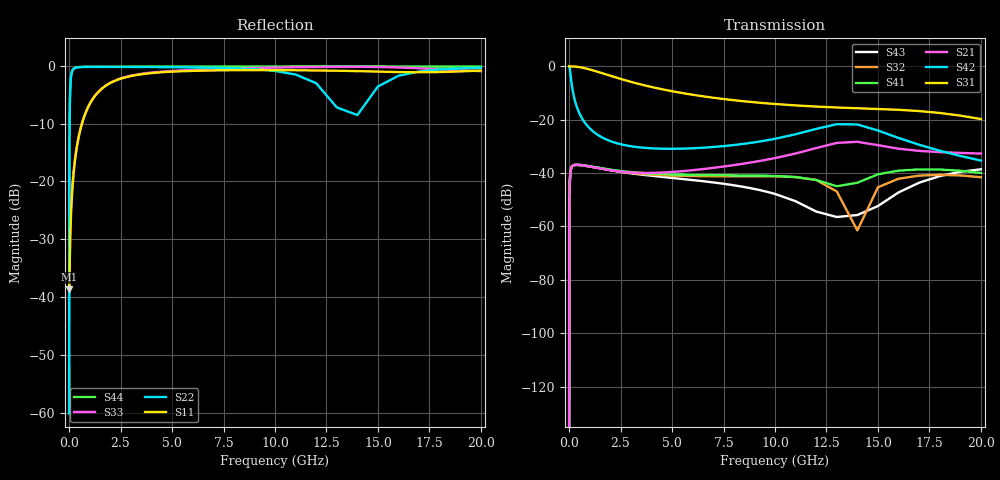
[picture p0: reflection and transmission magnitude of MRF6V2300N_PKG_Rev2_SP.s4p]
! Created Fri Apr 13 13:24:45 2007
# mhz S ma R 50
! 4 Port Network Data from SP1.SP block
! freq  magS11  angS11  magS12  angS12  magS13  angS13  magS14  angS14
!  magS21  angS21  magS22  angS22  magS23  angS23  magS24  angS24
!  magS31  angS31  magS32  angS32  magS33  angS33  magS34  angS34
!  magS41  angS41  magS42  angS42  magS43  angS43  magS44  angS44
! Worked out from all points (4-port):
!   1591 points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, 1 Hz to 20 GHz, reference 50 ohm
!   strongest paths, dB at 1 Hz, 267 MHz, 2.15 GHz, 6.13 GHz, 20 GHz:
!     S31: -0.1, -0.1, -4.0, -10.9, -19.8
!     S42: 0.0, -12.5, -28.5, -30.7, -35.4
!     S21: -193.0, -37.0, -39.2, -38.9, -32.7
!     S41: -193.0, -37.0, -38.9, -40.7, -40.0
!     S32: -192.8, -37.1, -39.1, -41.2, -41.6
!     S43: -192.8, -37.0, -39.2, -42.8, -38.6
!   lowest |S11| = -38.6 dB at 1.122 Hz (marker M1), VSWR 1.02, Z = 51.2 - j6.67e-08 ohm
!   |S11| at or under -10 dB: start of sweep to 626.5 MHz
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1e-06  0.01174 -0.0  2.241e-10 90.0  0.9883 -0.0  2.241e-10 90.0
       2.241e-10 90.0  0.000999 -0.0  2.289e-10 90.0  0.999 -0.0
       0.9883 -0.0  2.289e-10 90.0  0.01174 -0.0  2.299e-10 90.0
       2.241e-10 90.0  0.999 -0.0  2.299e-10 90.0  0.000999 -0.0
1.122097e-06  0.01174 -0.0  2.514e-10 90.0  0.9883 -0.0  2.514e-10 90.0
              2.514e-10 90.0  0.000999 -0.0  2.569e-10 90.0  0.999 -0.0
              0.9883 -0.0  2.569e-10 90.0  0.01174 -0.0  2.579e-10 90.0
              2.514e-10 90.0  0.999 -0.0  2.579e-10 90.0  0.000999 -0.0
4.508783  0.01201 -12.6  0.001008 86.0  0.9883 -0.1  0.001008 86.0
          0.001008 86.0  0.06755 -93.1  0.00103 85.9  0.9966 -3.9
          0.9883 -0.1  0.00103 85.9  0.01225 -18.1  0.001034 85.9
          0.001008 86.0  0.9966 -3.9  0.001034 85.9  0.06781 -93.1
28  0.01958 -55.4  0.005767 66.5  0.989 -0.7  0.005767 66.5
    0.005767 66.5  0.3861 -113.2  0.00587 65.8  0.9175 -22.8
    0.989 -0.7  0.00587 65.8  0.0242 -69.2  0.005894 65.9
    0.005767 66.5  0.9175 -22.8  0.005894 65.9  0.3876 -113.2
225  0.1206 -93.1  0.014 13.5  0.9871 -6.9  0.01401 13.2
     0.014 13.5  0.9374 -164.1  0.01392 12.3  0.278 -70.0
     0.9871 -6.9  0.01392 12.3  0.1269 -101.4  0.01398 12.8
     0.01401 13.2  0.278 -70.0  0.01398 12.8  0.9411 -163.9
3180  0.8233 -152.7  0.01011 -2.7  0.487 -57.5  0.01025 -13.1
      0.01011 -2.7  0.9731 177.2  0.009856 -17.0  0.03093 -47.3
      0.487 -57.5  0.009856 -17.0  0.8299 -153.0  0.009641 -10.7
      0.01025 -13.1  0.03093 -47.3  0.009641 -10.7  0.9795 -178.8
20000  0.9059 179.8  0.02306 107.8  0.1024 -143.8  0.01003 -58.3
       0.02306 107.8  0.957 -176.9  0.008327 -50.5  0.01708 -178.4
       0.1024 -143.8  0.008327 -50.5  0.8951 176.6  0.01172 110.3
       0.01003 -58.3  0.01708 -178.4  0.01172 110.3  0.9791 -179.8
